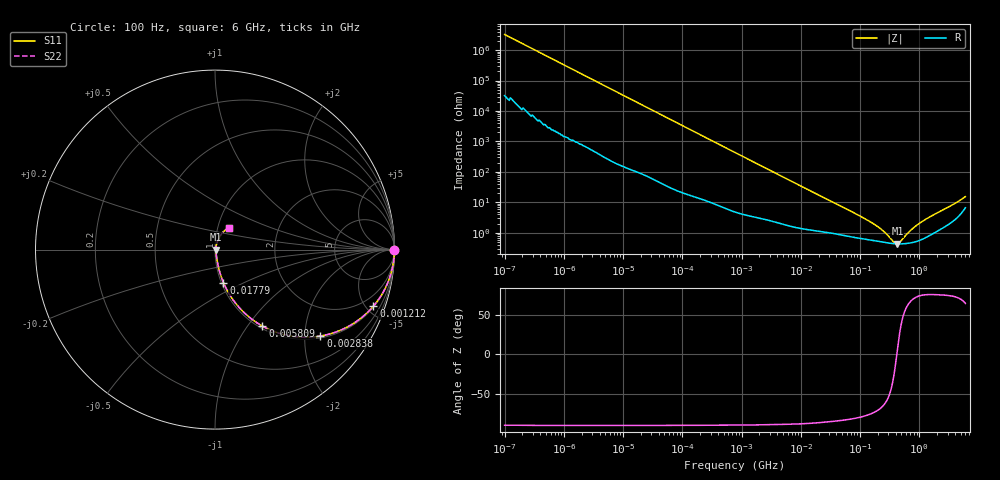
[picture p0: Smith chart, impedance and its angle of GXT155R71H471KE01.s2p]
!Murata Part Number: GXT155R71H471KE01
!These Parameters are Measured in Series Mode Connection
!Data Generated on Jan 08, 2026
!  o--ll--o
!Port1  Port2
!  o------o
!Operation Temp=25[degC], DC Bias Voltage=0[V]
!Freq. Start=100[Hz] Stop=6[GHz] 401[Steps]
# Hz S RI R 50
!Freq.(Hz) S11(Real) S11(Imag) S21(Real) S21(Imag) S12(Real) S12(Imag) S22(Real) S22(Imag)
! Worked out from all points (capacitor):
!   401 points, 100 Hz to 6 GHz, reference 50 ohm
!   read as one part in series: C = 487 pF near 109 Hz
!   lowest |Z| = 435 mohm at 427.4 MHz (marker M1)
!   series resonance near 416.8 MHz, so ESL is about 300 pH
!   S11 on the Smith chart (normalised r, x): 100 Hz: open; 1.212 MHz: 1.08, -5.56; 2.838 MHz: 1.05, -2.39; 5.809 MHz: 1.04, -1.18; 17.79 MHz: 1.02, -0.39; 6 GHz: 1.13, +0.28
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100  1 -3.06e-05  3e-07 3.06e-05  3e-07 3.06e-05  1 -3.06e-05
335  1 -0.000102  6e-07 0.000102  6e-07 0.000102  1 -0.000102
2008  1 -0.00061  3.3e-06 0.00061  3.3e-06 0.00061  1 -0.00061
40335  0.9998 -0.0121  0.000215 0.0121  0.000215 0.0121  0.9998 -0.0121
241822  0.9942 -0.0719  0.0058 0.0719  0.0058 0.0719  0.9942 -0.0719
774597  0.9475 -0.2176  0.0525 0.2176  0.0525 0.2176  0.9475 -0.2176
1212075  0.8822 -0.3157  0.1178 0.3157  0.1178 0.3157  0.8822 -0.3157
2837864  0.5868 -0.4817  0.4132 0.4817  0.4132 0.4817  0.5868 -0.4817
5809218  0.264 -0.4261  0.736 0.4261  0.736 0.4261  0.264 -0.4261
9090158  0.1345 -0.3227  0.8655 0.3227  0.8655 0.3227  0.1345 -0.3227
1.555665e7  0.0575 -0.2071  0.9425 0.2071  0.9425 0.2071  0.0575 -0.2071
1.779312e7  0.0469 -0.1836  0.9531 0.1836  0.9531 0.1836  0.0469 -0.1836
4.35672e7  0.0151 -0.0793  0.9849 0.0793  0.9849 0.0793  0.0151 -0.0793
1.395531e8  0.00645 -0.0238  0.9935 0.0238  0.9935 0.0238  0.00645 -0.0238
2.183701e8  0.00527 -0.0128  0.9947 0.0128  0.9947 0.0128  0.00527 -0.0128
3.124326e8  0.00459 -0.00559  0.9954 0.00559  0.9954 0.00559  0.00459 -0.00559
3.737127e8  0.00438 -0.00211  0.9956 0.00211  0.9956 0.00211  0.00438 -0.00211
4.274388e8  0.00431 0.000497  0.9957 -0.000497  0.9957 -0.000497  0.00431 0.000497
4.888888e8  0.00432 0.00313  0.9957 -0.00313  0.9957 -0.00313  0.00432 0.00313
7.31507e8  0.00482 0.0116  0.9952 -0.0116  0.9952 -0.0116  0.00482 0.0116
1.094528e9  0.00644 0.0219  0.9936 -0.0219  0.9936 -0.0219  0.00644 0.0219
6e9  0.0783 0.1209  0.9217 -0.1209  0.9217 -0.1209  0.0783 0.1209
